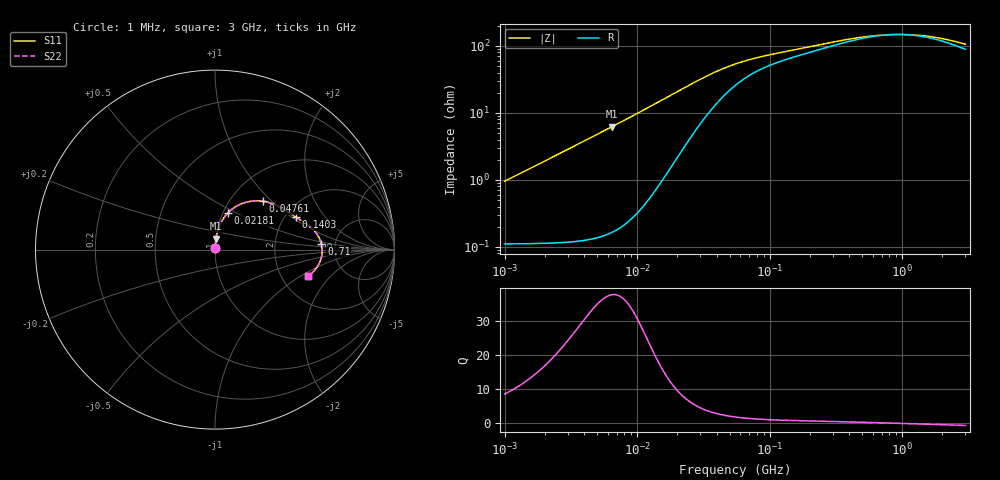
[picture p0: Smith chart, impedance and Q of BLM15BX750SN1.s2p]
! BLM15BX750SN1
# Hz S RI R 50
!Freq.(Hz) S11(Real) S11(Imag) S21(Real) S21(Imag) S12(Real) S12(Imag) S22(Real) S22(Imag)
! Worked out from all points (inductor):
!   401 points, 1 MHz to 3 GHz, reference 50 ohm
!   read as one part in series: L = 151 nH near 1.041 MHz
!   highest Q = 37.7 at 6.433 MHz (marker M1), where L = 153 nH
!   self-resonance near 912.6 MHz
!   S11 on the Smith chart (normalised r, x): 1 MHz: 1.00, +0.02; 21.81 MHz: 1.06, +0.45; 47.61 MHz: 1.40, +0.88; 140.3 MHz: 2.30, +1.08; 710 MHz: 3.88, +0.37; 3 GHz: 2.78, -1.15
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1000000  0.0012 0.00947  0.9988 -0.00947  0.9988 -0.00947  0.0012 0.00947
1083356  0.00121 0.0103  0.9988 -0.0103  0.9988 -0.0103  0.00121 0.0103
3823119  0.00256 0.0363  0.9974 -0.0363  0.9974 -0.0363  0.00256 0.0363
6433254  0.00544 0.0615  0.9946 -0.0615  0.9946 -0.0615  0.00544 0.0615
9992459  0.0126 0.0963  0.9874 -0.0963  0.9874 -0.0963  0.0126 0.0963
1.461624e7  0.0288 0.1414  0.9712 -0.1414  0.9712 -0.1414  0.0288 0.1414
2.181181e7  0.0716 0.2039  0.9284 -0.2039  0.9284 -0.2039  0.0716 0.2039
2.664524e7  0.1093 0.2353  0.8907 -0.2353  0.8907 -0.2353  0.1093 0.2353
3.254976e7  0.1585 0.2595  0.8415 -0.2595  0.8415 -0.2595  0.1585 0.2595
3.897472e7  0.209 0.2705  0.791 -0.2705  0.791 -0.2705  0.209 0.2705
4.761141e7  0.2653 0.2695  0.7347 -0.2695  0.7347 -0.2695  0.2653 0.2695
5.477226e7  0.3014 0.2618  0.6986 -0.2618  0.6986 -0.2618  0.3014 0.2618
8.173662e7  0.3816 0.2254  0.6184 -0.2254  0.6184 -0.2254  0.3816 0.2254
1.403209e8  0.4522 0.1798  0.5478 -0.1798  0.5478 -0.1798  0.4522 0.1798
2.094008e8  0.4967 0.1521  0.5033 -0.1521  0.5033 -0.1521  0.4967 0.1521
4.135554e8  0.5633 0.0931  0.4367 -0.0931  0.4367 -0.0931  0.5633 0.0931
7.099691e8  0.5927 0.0313  0.4073 -0.0313  0.4073 -0.0313  0.5927 0.0313
8.005644e8  0.5955 0.0165  0.4045 -0.0165  0.4045 -0.0165  0.5955 0.0165
1.10276e9  0.5959 -0.0242  0.4041 0.0242  0.4041 0.0242  0.5959 -0.0242
1.488926e9  0.5863 -0.0635  0.4137 0.0635  0.4137 0.0635  0.5863 -0.0635
2.092429e9  0.5611 -0.1076  0.4389 0.1076  0.4389 0.1076  0.5611 -0.1076
3e9  0.5156 -0.1476  0.4844 0.1476  0.4844 0.1476  0.5156 -0.1476
